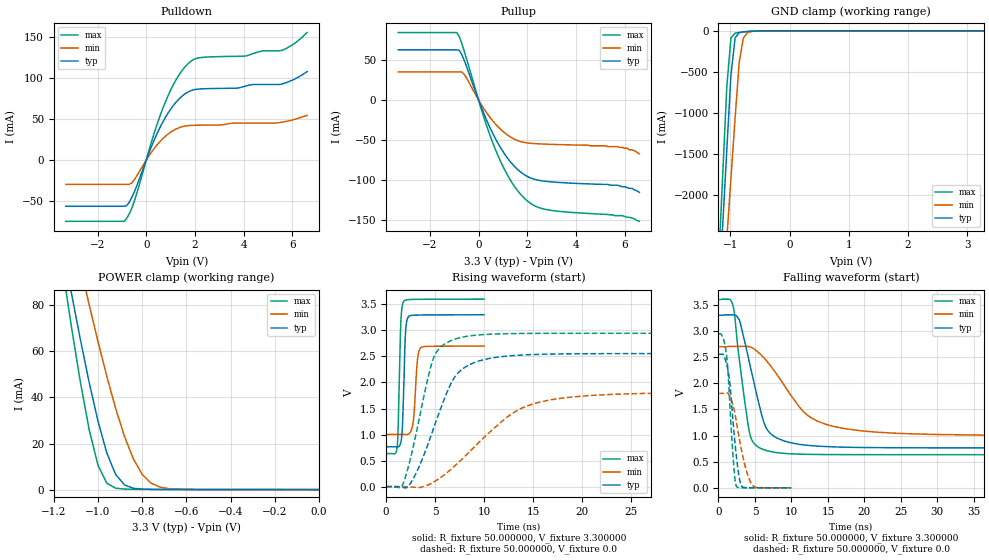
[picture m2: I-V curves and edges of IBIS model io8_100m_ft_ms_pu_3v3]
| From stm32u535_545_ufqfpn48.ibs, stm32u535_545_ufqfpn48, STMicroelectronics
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|   Model io8_100m_ft_ms_pu_3v3
[Model]  io8_100m_ft_ms_pu_3v3
Model_type I/O
Polarity   Non-Inverting
Enable   Active-Low
Vinl =   0.990000V
Vinh =   2.310000V
Vmeas =  1.650000V
Cref =   50.000000pF
Rref =   100.000000M
Vref =   0.0V
C_comp   3.313100pF   3.281800pF   3.354500pF
[Temperature Range]   25.000000   0.140000k   -40.000000
[Pullup Reference]   3.300000V   2.700000V   3.600000V
[Pulldown Reference]   0.0V   0.0V   0.0V
[POWER Clamp Reference]   3.300000V   2.700000V   3.600000V
[GND Clamp Reference]   0.0V   0.0V   0.0V
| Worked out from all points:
|   slope of the pulldown table from 0 to 0.495 V, typ, clamps not added: 14 ohm
|   slope of the pullup table from 0 to 0.495 V, typ, clamps not added: 13.7 ohm
|   GND clamp passes 1 mA (typ) near -0.51 V on its own axis
|   POWER clamp passes 1 mA (typ) near -0.85 V on its own axis
|   rising waveform, R_fixture 50.000000, V_fixture 3.300000: 20-80 % time 249ps typ, 340ps min, 234ps max; typ from 0.765 V to 3.3 V
|   rising waveform, R_fixture 50.000000, V_fixture 0.0: 20-80 % time 3.15ns typ, 6.44ns min, 2.09ns max; typ from 0.001 V to 2.55 V
|   falling waveform, R_fixture 50.000000, V_fixture 3.300000: 20-80 % time 2.58ns typ, 5.69ns min, 1.62ns max; typ from 3.3 V to 0.765 V
|   falling waveform, R_fixture 50.000000, V_fixture 0.0: 20-80 % time 1.01ns typ, 1.54ns min, 767ps max; typ from 2.55 V to 0.001 V
[Pulldown]
|Voltage   I(typ)   I(min)   I(max)
-3.3V     -56.06mA   -29.42mA   -74.35mA
-900mV    -56.06mA   -29.42mA   -74.35mA
-700mV    -51.09mA   -29.42mA   -65.48mA
-500mV    -39.32mA   -24.2mA    -50.88mA
300mV     22.62mA    13.13mA    30.42mA
800mV     52.54mA    29.36mA    71.75mA
1.3V      72.91mA    38.82mA    101.4mA
1.8V      84.02mA    42.13mA    119.4mA
2.3V      86.61mA    42.5mA     124.8mA
5.5V      91.97mA    45.76mA    132.8mA
6V        97.2mA     48.8mA     140mA
6.6V      107.6mA    54.5mA     155mA
[Pullup]
|Voltage   I(typ)   I(min)   I(max)
-3.3V     62.56mA    35.13mA    84.07mA
-900mV    62.56mA    35.13mA    84.07mA
-800mV    62.09mA    35.13mA    79.5mA
-600mV    50.25mA    32.46mA    61.91mA
200mV     -15.65mA   -9.933mA   -19.95mA
700mV     -48.51mA   -30.11mA   -62.22mA
1.3V      -76.68mA   -45.83mA   -99.4mA
1.6V      -86.41mA   -50.38mA   -112.8mA
2V        -95.1mA    -53.38mA   -125.6mA
2.8V      -101.3mA   -54.97mA   -136.5mA
5.7V      -106mA     -58mA      -144mA
6.6V      -115mA     -67mA      -151mA
[GND_clamp]
|Voltage   I(typ)   I(min)   I(max)
-3.3V     -9.848A    -9.957A    -9.458A
-1.2V     -3.312A    -4.013A    -2.863A
-1.13V    -2.381A    -3.274A    -1.769A
-1.06V    -1.452A    -2.535A    -684.7mA
-990mV    -542.9mA   -1.798A    -88.02mA
-920mV    -87.11mA   -1.064A    -28.44mA
-850mV    -22.1mA    -382.4mA   -19.61mA
-780mV    -11.97mA   -86.98mA   -13.71mA
-710mV    -7.619mA   -22.26mA   -8.745mA
-640mV    -4.493mA   -7.773mA   -4.817mA
-360mV    -31.22uA   -172.6uA   -8.607uA
3.28V     0A         15.66nA    -5.841nA
[POWER_clamp]
|Voltage   I(typ)   I(min)   I(max)
-3.28V    1.355A     1.167A     1.665A
-1.16V    105.8mA    131.6mA    95.87mA
-1.12V    85.08mA    114mA      70.45mA
-1.08V    65.19mA    96.88mA    46.75mA
-1.04V    46.48mA    80.2mA     25.96mA
-1V       29.64mA    64.18mA    10.49mA
-960mV    15.81mA    49.06mA    2.743mA
-920mV    6.481mA    35.16mA    612.9uA
-840mV    578.2uA    13.29mA    138.5uA
-760mV    94.37uA    2.807mA    98.56uA
-640mV    40.55uA    159.2uA    59.96uA
0V        0A         19.29nA    0A
[Ramp]
| variable   typ   min   max
dV/dt_r  1.53214/3.14687n   1.08405/6.43063n   1.76624/2.08585n
dV/dt_f  1.52095/2.57342n   1.01826/5.67592n   1.77907/1.61727n
R_load = 50.000000
[Rising Waveform]
R_fixture= 50.000000
V_fixture= 3.300000
V_fixture_min= 2.700000
V_fixture_max= 3.600000
|time   V(typ)   V(min)   V(max)
0s        765.1mV    1.003V     634.9mV
1.121ns   762.2mV    1.003V     758.7mV
1.502ns   854.6mV    1.003V     3.163V
1.782ns   1.822V     1.002V     3.555V
1.982ns   2.974V     1V         3.581V
2.262ns   3.259V     1.008V     3.589V
2.763ns   3.29V      1.247V     3.595V
3.163ns   3.293V     2.371V     3.596V
3.524ns   3.295V     2.664V     3.597V
9.97ns    3.3V       2.7V       3.6V
[Rising Waveform]
R_fixture= 50.000000
V_fixture= 0.0
V_fixture_min= 0.0
V_fixture_max= 0.0
|time   V(typ)   V(min)   V(max)
0s        835.9uV    853.7uV    880.3uV
1.562ns   -12.49mV   908.8uV    -10.85mV
2.523ns   74.28mV    -6.078mV   571.5mV
4.805ns   1.102V     83.1mV     2.455V
6.486ns   1.93V      311.9mV    2.792V
7.568ns   2.225V     497.4mV    2.861V
9.489ns   2.414V     854mV      2.913V
13.09ns   2.518V     1.431V     2.939V
17.66ns   2.547V     1.692V     2.944V
59.82ns   2.554V     1.808V     2.945V
[Falling Waveform]
R_fixture= 50.000000
V_fixture= 3.300000
V_fixture_min= 2.700000
V_fixture_max= 3.600000
|time   V(typ)   V(min)   V(max)
0s        3.3V       2.7V       3.6V
1.922ns   3.308V     2.706V     3.516V
2.162ns   3.307V     2.706V     3.364V
2.883ns   3.198V     2.706V     2.423V
4.444ns   2.265V     2.689V     958.4mV
6.486ns   1.16V      2.446V     717mV
8.168ns   942.6mV    2.135V     672.2mV
12.13ns   815.3mV    1.396V     641.9mV
17.3ns    778.4mV    1.133V     636.3mV
59.82ns   765.1mV    1.003V     634.9mV
[Falling Waveform]
R_fixture= 50.000000
V_fixture= 0.0
V_fixture_min= 0.0
V_fixture_max= 0.0
|time   V(typ)   V(min)   V(max)
0s        2.554V     1.808V     2.945V
640.6ps   2.549V     1.808V     2.86V
1.101ns   2.377V     1.81V      2.536V
1.542ns   2.023V     1.752V     1.629V
2.042ns   1.194V     1.555V     513.5mV
2.442ns   616.3mV    1.273V     36.46mV
3.123ns   47.97mV    743.2mV    3.442mV
3.904ns   4.167mV    293.7mV    2.126mV
4.745ns   2.347mV    40.58mV    1.653mV
9.97ns    835.9uV    853.7uV    880.3uV
